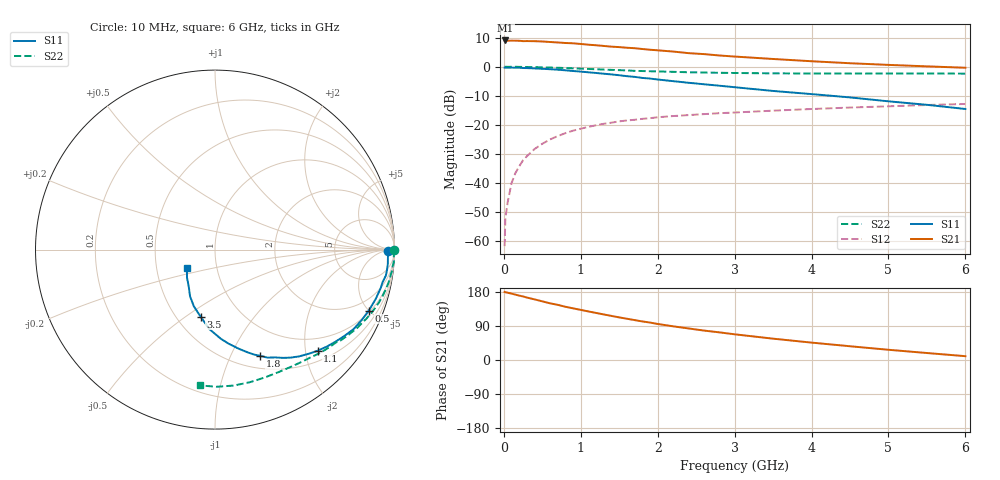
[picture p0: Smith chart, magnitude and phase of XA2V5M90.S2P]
! SIEMENS Discrete & RF Semiconductors
! BFY180
! Si NPN RF Bipolar Junction Transistor in MICRO-X
! VCE = 2.5 V  IC = 0.9 mA
! Common Emitter S-Parameters:  May  1997
# GHz  S  MA  R  50
!  f  S11  S21  S12  S22
! GHz  MAG  ANG  MAG  ANG  MAG  ANG  MAG  ANG
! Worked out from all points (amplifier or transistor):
!   36 points, 10 MHz to 6 GHz, reference 50 ohm
!   highest |S21| = 9.1 dB at 20 MHz (marker M1)
!   |S21| within 3 dB of that: start of sweep to 1.82 GHz
!   unconditionally stable (mu >= 1): 3.934 GHz to end of sweep
!   at 250 MHz: K = 0.06, MSG = 20.5 dB, |S12| = -32.3 dB
!   at 1.4 GHz: K = 0.49, MSG = 13.1 dB, |S12| = -19.3 dB
!   at 6 GHz: K = 1.06, MAG = 4.8 dB, |S12| = -12.8 dB
!   S11 on the Smith chart (normalised r, x): 10 MHz: 55, -11; 500 MHz: 1.11, -5.01; 1.1 GHz: 0.71, -2.25; 1.8 GHz: 0.64, -1.30; 3.5 GHz: 0.65, -0.57; 6 GHz: 0.72, -0.15
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0.01  0.9657 -0.4  2.8 179.6  0.0008 94.3  0.9981 -0.2
0.02  0.9633 -0.9  2.844 178.8  0.0024 89.0  0.9999 -0.5
0.05  0.9641 -1.9  2.813 177.6  0.0046 82.9  0.9964 -1.2
0.1  0.9662 -4.6  2.822 175.1  0.0098 86.5  0.9974 -2.6
0.15  0.9651 -6.8  2.819 172.6  0.0146 86.3  0.9982 -4.0
0.25  0.9507 -11.1  2.768 167.7  0.0244 83.3  0.9941 -6.7
0.4  0.9363 -17.2  2.763 159.9  0.0381 77.3  0.9853 -10.4
0.5  0.9219 -21.6  2.732 154.8  0.0468 74.2  0.9775 -12.9
0.6  0.9071 -25.6  2.676 149.6  0.0556 71.6  0.9696 -15.3
0.8  0.868 -33.5  2.571 140.5  0.0714 66.3  0.9499 -20.0
0.9  0.8451 -37.4  2.54 136.3  0.0789 63.4  0.9382 -22.3
1.1  0.8026 -44.6  2.402 128.1  0.0917 58.6  0.916 -26.4
1.5  0.7138 -57.7  2.184 112.4  0.1141 50.1  0.8735 -34.1
1.8  0.6418 -67.1  2.025 101.8  0.1261 45.6  0.8433 -39.0
2.2  0.5645 -77.0  1.831 88.9  0.1409 39.6  0.817 -45.3
2.6  0.4991 -86.1  1.654 77.7  0.1522 35.2  0.7946 -50.8
3  0.4434 -94.1  1.5 67.8  0.1622 31.0  0.7804 -56.1
3.5  0.3822 -102.1  1.362 56.3  0.1747 26.9  0.7692 -62.4
4  0.3375 -110.4  1.245 45.9  0.1865 22.7  0.7647 -68.8
4.5  0.2958 -118.0  1.15 36.3  0.1976 18.8  0.764 -75.4
5.5  0.2203 -135.1  1.016 18.4  0.2187 10.9  0.7642 -89.2
6  0.1866 -146.8  0.961 10.1  0.2279 6.8  0.7615 -96.2
